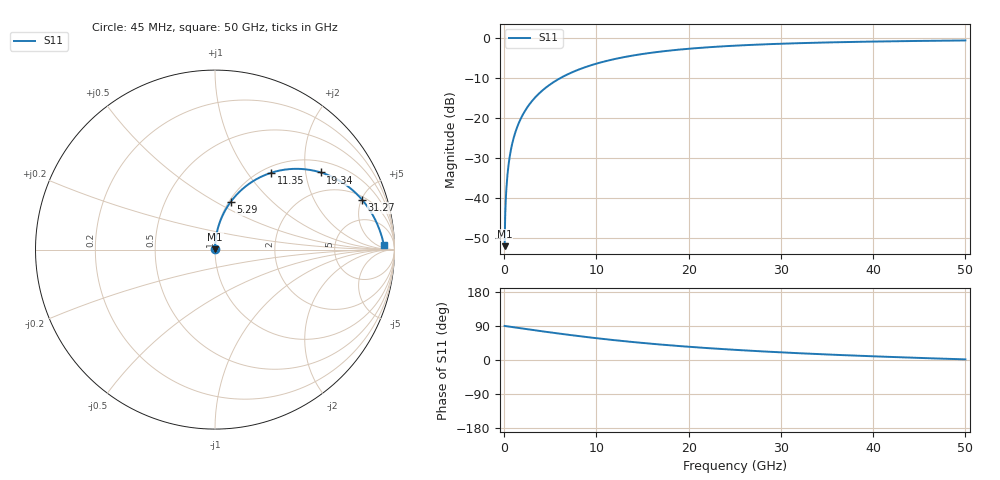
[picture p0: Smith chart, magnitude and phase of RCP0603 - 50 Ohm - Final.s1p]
!Vishay Electro-Films Inc.
!RCP Family
!Case Size 0603
!Assembly Style Surface Mount
!11/2/2015
!efi@vishay.com
# GHz S MA R 50
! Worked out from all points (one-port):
!   801 points, 45 MHz to 50 GHz, reference 50 ohm
!   lowest |S11| = -52.1 dB at 45 MHz (marker M1), VSWR 1.00, Z = 50 + j0.247 ohm
!   |S11| at or under -10 dB: start of sweep to 6.062 GHz
!   S11 on the Smith chart (normalised r, x): 45 MHz: 1.00, +0.00; 5.29 GHz: 1.02, +0.59; 11.35 GHz: 1.10, +1.30; 19.34 GHz: 1.32, +2.43; 31.27 GHz: 2.30, +5.07; 50 GHz: 27, +13
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0.045  0.002474 89.8
0.1698875  0.009339 89.4
0.3572187  0.01963 88.7
0.4196625  0.02307 88.5
0.54455  0.02992 88.1
0.6694375  0.03678 87.6
0.8567687  0.04705 87.0
1.0441  0.05731 86.3
1.293875  0.07095 85.5
1.606094  0.08796 84.4
1.980756  0.1083 83.1
2.417863  0.1318 81.5
2.854969  0.1551 80.0
3.978956  0.2137 76.2
5.290275  0.2793 71.8
6.289375  0.3268 68.6
8.599794  0.4275 61.5
11.34732  0.5295 53.9
12.53375  0.5677 50.8
15.40616  0.6468 44.1
18.77812  0.7189 37.2
19.34012  0.7291 36.1
22.15009  0.7736 31.2
25.0225  0.8098 26.8
31.26687  0.8655 18.7
37.51125  0.901 12.1
43.75563  0.9247 6.5
50  0.9411 1.7
